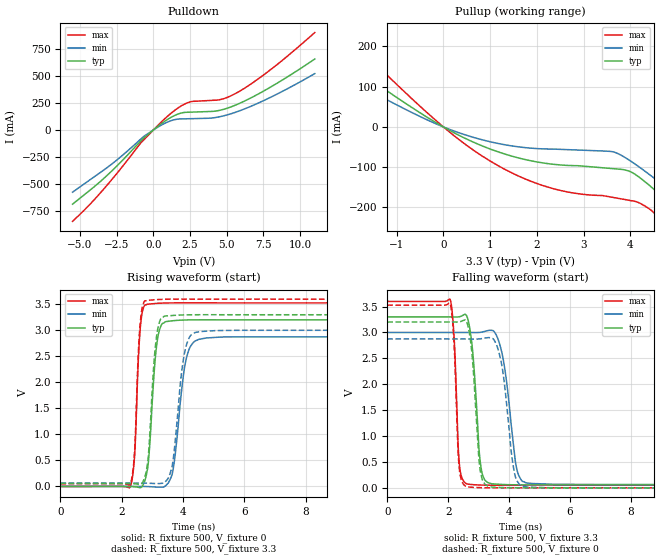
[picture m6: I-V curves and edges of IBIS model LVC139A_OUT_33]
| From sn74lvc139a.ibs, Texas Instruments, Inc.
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[Model]   LVC139A_OUT_33
Model_type  Output
Vref =   0
Rref =   500
Cref =   50p
Vmeas =   1.5
| variable   typ   min   max
C_comp   5.36pF   2.63pF   9.30pF
| C_pullup   4.81pF   3.25pF   7.45pF
| C_pulldown   5.90pF   2.63pF   9.30pF
[Temperature Range]   40   100   -40
| Ambient temperature   25   85   -40
[Voltage range]   3.3   3   3.6
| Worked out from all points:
|   slope of the pulldown table from 0 to 0.495 V, typ, clamps not added: 9.22 ohm
|   slope of the pullup table from 0 to 0.495 V, typ, clamps not added: 16.5 ohm
|   rising waveform, R_fixture 500, V_fixture 0: 20-80 % time 216ps typ, 317ps min, 145ps max; typ from 0 V to 3.2 V
|   falling waveform, R_fixture 500, V_fixture 3.3: 20-80 % time 218ps typ, 351ps min, 137ps max; typ from 3.3 V to 0.057 V
|   rising waveform, R_fixture 500, V_fixture 3.3: 20-80 % time 208ps typ, 299ps min, 143ps max; typ from 0.057 V to 3.3 V
|   falling waveform, R_fixture 500, V_fixture 0: 20-80 % time 214ps typ, 318ps min, 134ps max; typ from 3.2 V to 0 V
[Pulldown]
| LVC139A_OUT_33
|   Voltage   I(typ)   I(min)   I(max)
-5.5V     -685.5mA   -574.6mA   -843.9mA
-3.485V   -461.2mA   -380.8mA   -562.8mA
-2.265V   -302.9mA   -252.4mA   -364.9mA
-600mV    -67.64mA   -54.33mA   -84.08mA
550mV     59.31mA    46.12mA    75.08mA
1.375V    129.6mA    93.32mA    173.3mA
1.935V    158.4mA    103.2mA    225.8mA
2.475V    165.2mA    104.9mA    259.1mA
4.535V    183mA      123.4mA    281.1mA
5.715V    237.5mA    170.1mA    346.7mA
8.05V     402.3mA    307.1mA    564.9mA
11V       657.2mA    522mA      901.7mA
[Pullup]
| LVC139A_OUT_33
|   Voltage   I(typ)   I(min)   I(max)
-5.5V     468.7mA    372.3mA    650.8mA
-4.01V    330.8mA    259.6mA    462.9mA
-3.12V    251mA      195.1mA    353.4mA
-2.31V    180.7mA    138.9mA    256.2mA
1.02V     -55.72mA   -37.37mA   -86.09mA
2.24V     -91.25mA   -54.88mA   -149.7mA
3.625V    -103.6mA   -61.73mA   -175.1mA
4.225V    -128.1mA   -102.6mA   -190.8mA
4.81V     -186.7mA   -154.6mA   -250.4mA
5.28V     -237.9mA   -198.8mA   -312.7mA
5.875V    -304.8mA   -256mA     -395.1mA
11V       -910mA     -769.5mA   -1.146A
[Ramp]
| LVC139A_OUT_33
| variable   typ   min   max
dV/dt_r   1.94/2.28E-10   1.73/3.37E-10   2.13/1.48E-10
dV/dt_f   1.98/2.30E-10   1.79/3.66E-10   2.16/1.42E-10
R_load = 500
[Rising Waveform]
| LVC139A_OUT_33
R_fixture =   500
C_fixture =   0
L_fixture =   0
V_fixture =   0
V_fixture_min = 0
V_fixture_max = 0
|   Time   V(typ)   V(min)   V(max)
0s        30.63pV    2.102nV    1.768nV
2.28ns    -13.04uV   -35.56uV   -1.135mV
2.425ns   -6.516mV   102.1uV    637.7mV
2.61ns    -23.89mV   583.6uV    3.084V
2.84ns    335.5mV    -2.21mV    3.504V
3.165ns   2.827V     -14.05mV   3.52V
3.575ns   3.18V      130mV      3.528V
4.115ns   3.2V       2.483V     3.529V
4.765ns   3.203V     2.854V     3.529V
50ns      3.202V     2.874V     3.528V
[Falling Waveform]
| LVC139A_OUT_33
R_fixture =   500
C_fixture =   0
L_fixture =   0
V_fixture =   3.3
V_fixture_min = 3
V_fixture_max = 3.6
|   Time   V(typ)   V(min)   V(max)
0s        3.3V       3V         3.6V
2.065ns   3.3V       3V         3.638V
2.2ns     3.3V       3V         2.861V
2.37ns    3.304V     3V         446.6mV
2.68ns    3.176V     3V         68.45mV
3.07ns    435.3mV    3.004V     54.16mV
3.435ns   78.81mV    3.04V      50.47mV
4.26ns    58.29mV    353.8mV    49.78mV
4.595ns   56.9mV     92.52mV    49.9mV
50ns      56.71mV    64.25mV    50.1mV
[Rising Waveform]
| LVC139A_OUT_33
R_fixture =   500
C_fixture =   0
L_fixture =   0
V_fixture =   3.3
V_fixture_min = 3
V_fixture_max = 3.6
|   Time   V(typ)   V(min)   V(max)
0s        56.71mV    64.25mV    50.1mV
2.28ns    56.63mV    64.22mV    52.62mV
2.42ns    50.89mV    64.34mV    688.3mV
2.605ns   37.58mV    64.76mV    3.165V
2.84ns    440.9mV    62.08mV    3.58V
3.245ns   3.186V     56.41mV    3.595V
3.645ns   3.285V     392.5mV    3.6V
4.095ns   3.298V     2.692V     3.601V
4.57ns    3.301V     2.977V     3.6V
50ns      3.3V       3V         3.6V
[Falling Waveform]
| LVC139A_OUT_33
R_fixture =   500
C_fixture =   0
L_fixture =   0
V_fixture =   0
V_fixture_min = 0
V_fixture_max = 0
|   Time   V(typ)   V(min)   V(max)
0s        3.202V     2.874V     3.528V
2.065ns   3.202V     2.874V     3.559V
2.36ns    3.205V     2.874V     412.1mV
2.67ns    3.075V     2.874V     15.72mV
3.05ns    355.3mV    2.877V     3.575mV
3.43ns    14.95mV    2.89V      254.8uV
3.775ns   5.615mV    2.333V     -321uV
4.195ns   1.015mV    249.2mV    -302.8uV
4.6ns     -60.93uV   15.46mV    -167.9uV
50ns      -1.616nV   -1.975nV   2.984nV
